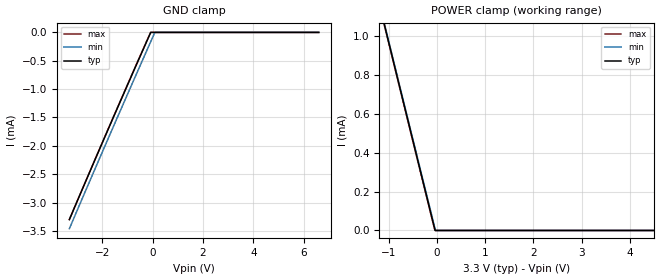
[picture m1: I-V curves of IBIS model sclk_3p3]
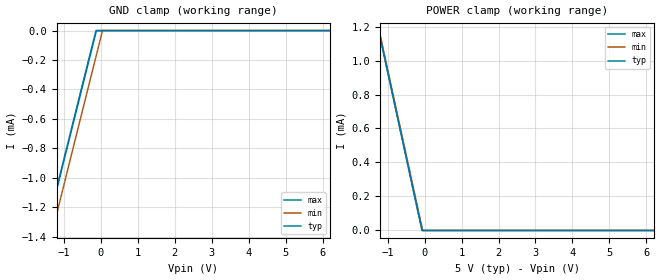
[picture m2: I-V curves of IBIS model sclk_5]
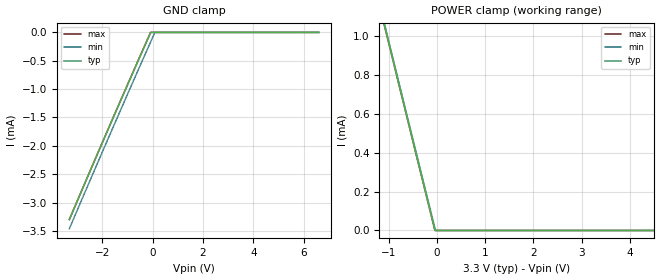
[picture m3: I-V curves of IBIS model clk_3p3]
|Texas Instruments Incorporated
| 24-bit, 240SPS ADC with 4-ch Diff Input Mux, High-Z Buffer, Serial Output
| Marketing part#   Digital Voltage Range   Package-type   #pins
| ADS1224IPWR   2.7V  - 5.5V   TSSOP   20
| ADS1224IPWRG4   2.7V  - 5.5V   TSSOP   20
| ADS1224IPWT   2.7V  - 5.5V   TSSOP   20
| ADS1224IPWTG4   2.7V  - 5.5V   TSSOP   20
[IBIS Ver]   3.2
[File name]   ads1224.ibs
|SIMDE Ver   V2.2 - 201009 - RHL4 - Build 424
[File Rev]   1.0
[Date]   8/29/2011
[Source]
| Texas Instruments Incorporated.
| Analog-eLab Design Center, HPA
| 12500 TI Blvd
| Dallas, TX -75243
| e-mail: elab_scm_ibis@list.ti.com
[Notes]   Revision History:
| Rev 1.0: 8/29/2011
| - Initial version of the model
| - Model generated from simulations in SPECTRE
| - Model matched to SPICE simulation
| - C_comp although listed in numerical order of value are
|   obtained from varying PVT conditions. For PVT conditions for
|   each specific value refer the buffer description under
|   respective [Model]. IBIS model user is responsible for using
|   appropriate C_comp to simulate for Signal Integrity.
| - Model names with a trailing _3p3 contains the model for
|   3.3V [3.0V and 3.6V]. Model names with a trailing _5 contains
|   the model for 5.0V [4.5V and 5.5V].
| - This is the Relative part of ADS1222.
|*  EXCEPTION:   *
|*  - For model sclk_* and clk_*, there is a small leakage current   *
|*   in the GND clamp I-V Table MIN corner because of a diode (D0)   *
|*   connected to the PAD.   *
|*  - For model bufen_*, there will be a leakage current in the POWER   *
|*   clamp I-V Table because of the pulldown on pad.   *
|*  - For model mux_tempen_*, there will be a small leakage current   *
|*   in the GND clamp I-V Table MIN corner because of a diode (D0)   *
|*   connected to pad.   *
[Disclaimer]
| This model is designed as an aid for customers of Texas Instruments.
| TI and its licensors and suppliers make no warranties, either expressed
| or implied, with respect to this  model, including the warranties of
| merchantability or fitness for a particular purpose. The model is
| provided solely on an "as is" basis. The entire risk as to its quality
| and performance is with the customer.
[Copyright]
 (C) Copyright 2011 Texas Instruments Incorporated.All rights reserved.
|   ADS1224PW
[Component]   ADS1224PW
[Manufacturer]   TI
[Package]   |20 TSSOP  -  PW package
|   typ   min   max
R_pkg   0.044165   0.01667   0.06355
L_pkg   2.231049nH   1.30214nH   3.55562nH
C_pkg   0.3357835pF  0.26626pF   0.48543pF
[Pin]  signal_name   model_name   R_pin   L_pin   C_pin
1   DVDD   POWER   0.01363   2.18216nH  0.49716pF
2   SCLK   SCLK   0.04443   2.52681nH  0.38913pF
3   CLK   CLK   0.036   1.70427nH  0.27091pF
4   _DRDY/DOUT   DRDY_DOUT   0.0384   1.7807nH   0.27673pF
5   MUX0   MUX_TEMPEN   0.03699   1.73537nH  0.27583pF
6   MUX1   MUX_TEMPEN   0.03229   1.5862nH   0.26626pF
7   TEMPEN   MUX_TEMPEN   0.04004   1.83871nH  0.28493pF
8   BUFEN   BUFEN   0.0517   2.22732nH  0.30833pF
9   AINP4   TERM   0.06355   3.17175nH  0.43038pF
10   AINN4   TERM   0.06313   3.55562nH  0.48543pF
11   AINP3   TERM   0.06289   3.54788nH  0.48475pF
12   AINN3   TERM   0.06313   3.16231nH  0.42865pF
13   AINP2   TERM   0.05073   2.195nH   0.30617pF
14   AINN2   TERM   0.03899   1.80445nH  0.28204pF
15   AINP1   TERM   0.01667   1.30214nH  0.29173pF
16   AINN1   TERM   0.03284   1.60803nH  0.2669pF
17   GND   GND   0.03147   1.56147nH  0.26508pF
18   VREFN   TERM   0.03505   1.67383nH  0.27069pF
19   VREFP   TERM   0.04397   2.50745nH  0.38946pF
20   AVDD   POWER   0.04589   2.96865nH  0.44887pF
|   Model Selectors
[Model Selector] SCLK
sclk_3p3   3.3V digital input
sclk_5   5.0V digital input
[Model Selector] CLK
clk_3p3   3.3V digital input
clk_5   5.0V digital input
[Model Selector] BUFEN
bufen_3p3  3.3V digital input
bufen_5   5.0V digital input
[Model Selector] MUX_TEMPEN
mux_tempen_3p3  3.3V digital input
mux_tempen_5   5.0V digital input
[Model Selector] DRDY_DOUT
drdy_dout_3p3   3.3V digital output
drdy_dout_5   5.0V digital output
[Model Selector] TERM
term_3-3V  3.3V nominal termination
term_5-0V  5.0V nominal termination
[Model] term_3-3V
Model_type Terminator
C_comp   1.0e-20F  1.0e-20F  1.0e-20F
|   typ   min   max
[Voltage Range]   3.3V   3.0V   3.6V
[POWER Clamp Reference]   3.3V   3.0V   3.6V
[GND Clamp Reference]   0V   0V   0V
|Ambient Temperature   25   85   -40
|Junction Temperature
[Temperature Range]   25   85   -40
[Model] term_5-0V
Model_type Terminator
C_comp   1.0e-20F  1.0e-20F  1.0e-20F
|   typ   min   max
[Voltage Range]   5.0V   4.5V   5.5V
[POWER Clamp Reference]   5.0V   4.5V   5.5V
[GND Clamp Reference]   0V   0V   0V
|Ambient Temperature   25   85   -40
|Junction Temperature
[Temperature Range]   25   85   -40
| Models and submodels in the file (12): sclk_3p3 (Input), sclk_5 (Input), clk_3p3 (Input), clk_5 (Input), bufen_3p3 (Input), bufen_5 (Input), mux_tempen_3p3 (Input), mux_tempen_5 (Input), drdy_dout_3p3 (Output), drdy_dout_5 (Output), term_3-3V (Terminator), term_5-0V (Terminator)
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|   sclk_3p3 Model
[Model]   sclk_3p3
Model_type   Input
Vinl = 0.66
Vinh = 2.64
|   typ   min   max
|   (nom PVT)   (fast PVT)   (slow PVT)
|C_comp from frequency sweep method (F= 5MHz)
|Average
C_comp   2.052e-15   1.706e-15   2.457e-15
|C_comp from LC tank measurement(L=1nH)
|Average
|resonant Frequency(Hz)   1.000e+12   1.000e+12   1.000e+12
|C_comp   2.536e-17   2.536e-17   2.536e-17
[Model spec]
Vinl   0.66   0.6   0.72
Vinh   2.64   2.4   2.88
| Where nom  PVT is Nominal Process, 3.3V, 25C
|   Fast PVT is Strong Process,  3.6V, -40C
|   Slow PVT is Weak Process,   3V, 85C
[Voltage Range]   3.3   3   3.6
|Ambient Temperature   25   85   -40
|Junction Temperature
[Temperature Range]   25   85   -40
[Power Clamp Reference]   3.3   3   3.6
[GND Clamp Reference]   0   0   0
[GND Clamp]
|   Voltage   I(typ)   I(min)   I(max)
-3.3V     -3.299mA   -3.46mA    -3.299mA
-1.756V   -1.703mA   -1.867mA   -1.698mA
-81.6mV   -10.64uA   -174.8uA   -3.025uA
93mV      0A         0A         0A
6.6V      0A         0A         0A
[POWER Clamp]
|   Voltage   I(typ)   I(min)   I(max)
-3.3V     3.297mA    3.298mA    3.297mA
-1.136V   1.098mA    1.104mA    1.094mA
-825mV    784.3uA    790.6uA    780uA
-49.2mV   6.178uA    14.35uA    1.715uA
-42mV     1.155uA    7.161uA    0A
-30mV     0A         0A         0A
6.6V      0A         0A         0A
|   sclk_5 Model
[Model]   sclk_5
Model_type   Input
Vinl = 1
Vinh = 4
|   typ   min   max
|   (nom PVT)   (fast PVT)   (slow PVT)
|C_comp from frequency sweep method (F= 5MHz)
|Average
C_comp   2.384e-15   1.992e-15   2.857e-15
|C_comp from LC tank measurement(L=1nH)
|Average
|resonant Frequency(Hz)   1.000e+12   1.000e+12   1.000e+12
|C_comp   2.536e-17   2.536e-17   2.536e-17
[Model spec]
Vinl   1   0.9   1.1
Vinh   4   3.6   4.4
| Where nom  PVT is Nominal Process, 5V, 25C
|   Fast PVT is Strong Process,  5.5V, -40C
|   Slow PVT is Weak Process,   4.5V, 85C
[Voltage Range]   5   4.5   5.5
|Ambient Temperature   25   85   -40
|Junction Temperature
[Temperature Range]   25   85   -40
[Power Clamp Reference]   5   4.5   5.5
[GND Clamp Reference]   0   0   0
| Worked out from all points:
|   GND clamp passes 1 mA (typ) near -1.12 V on its own axis
|   POWER clamp passes 1 mA (typ) near -1.06 V on its own axis
[GND Clamp]
|   Voltage   I(typ)   I(min)   I(max)
-5V       -4.998mA   -5.159mA   -4.998mA
-1.728V   -1.621mA   -1.785mA   -1.609mA
-1.25V    -1.136mA   -1.301mA   -1.124mA
-226mV    -105.9uA   -270.6uA   -93.46uA
-138mV    -17.71uA   -182.5uA   -5.421uA
-127mV    -6.705uA   -171.5uA   0A
-115mV    0A         -159.5uA   0A
40mV      0A         0A         0A
10V       0A         0A         0A
[POWER Clamp]
|   Voltage   I(typ)   I(min)   I(max)
-5V       4.996mA    4.997mA    4.996mA
-1.247V   1.185mA    1.195mA    1.179mA
-1.106V   1.043mA    1.053mA    1.037mA
-72mV     6.562uA    19.92uA    290.4nA
-54.5mV   0A         2.47uA     0A
-45.5mV   0A         0A         0A
10V       0A         0A         0A
|   clk_3p3 Model
[Model]   clk_3p3
Model_type   Input
Vinl = 0.66
Vinh = 2.64
|   typ   min   max
|   (nom PVT)   (fast PVT)   (slow PVT)
|C_comp from frequency sweep method (F= 8MHz)
|Average
C_comp   8.016e-16   6.665e-16   9.597e-16
|C_comp from LC tank measurement(L=1nH)
|Average
|Resonant Frequency(Hz)   1.000e+12   1.000e+12   1.000e+12
|C_comp   2.536e-17   2.536e-17   2.536e-17
[Model spec]
Vinl   0.66   0.6   0.72
Vinh   2.64   2.4   2.88
| Where nom  PVT is Nominal Process, 3.3V, 25C
|   Fast PVT is Strong Process,  3.6V, -40C
|   Slow PVT is Weak Process,   3V, 85C
[Voltage Range]   3.3   3   3.6
|Ambient Temperature   25   85   -40
|Junction Temperature
[Temperature Range]   25   85   -40
[Power Clamp Reference]   3.3   3   3.6
[GND Clamp Reference]   0   0   0
[GND Clamp]
|   Voltage   I(typ)   I(min)   I(max)
-3.3V     -3.299mA   -3.46mA    -3.299mA
-1.756V   -1.703mA   -1.867mA   -1.698mA
-81.6mV   -10.64uA   -174.8uA   -3.025uA
93mV      0A         0A         0A
6.6V      0A         0A         0A
[POWER Clamp]
|   Voltage   I(typ)   I(min)   I(max)
-3.3V     3.297mA    3.298mA    3.297mA
-1.136V   1.098mA    1.104mA    1.094mA
-825mV    784.3uA    790.6uA    780uA
-49.2mV   6.178uA    14.35uA    1.715uA
-42mV     1.155uA    7.161uA    0A
-30mV     0A         0A         0A
6.6V      0A         0A         0A
